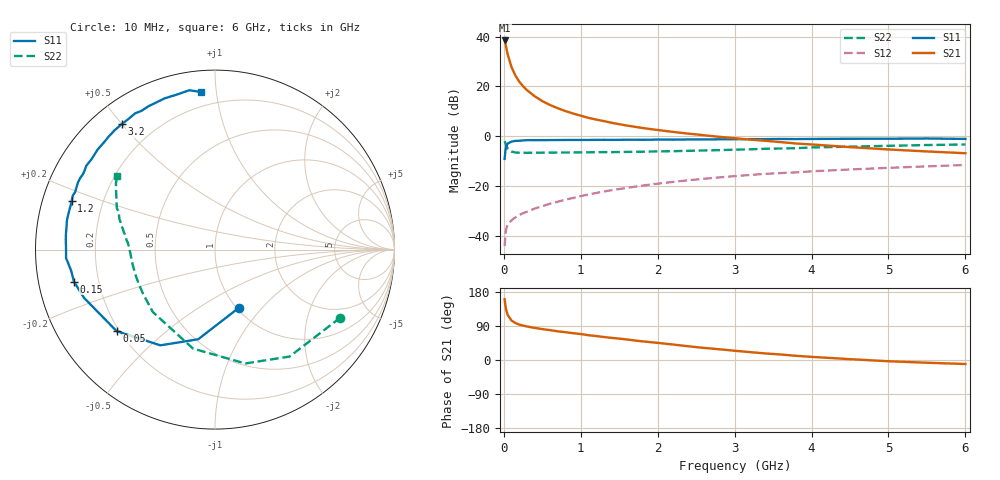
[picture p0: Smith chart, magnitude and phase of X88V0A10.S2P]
! SIEMENS Small Signal Semiconductors
! BFP136W
! Si NPN RF Bipolar Junction Transistor in SOT343
! VCE = 8 V  IC = 100 mA
! Common Emitter S-Parameters:  September  1994
# GHz  S  MA  R  50
!  f  S11  S21  S12  S22
! GHz  MAG  ANG  MAG  ANG  MAG  ANG  MAG  ANG
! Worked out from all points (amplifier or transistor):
!   40 points, 10 MHz to 6 GHz, reference 50 ohm
!   highest |S21| = 38.4 dB at 10 MHz (marker M1)
!   |S21| within 3 dB of that: start of sweep to 31.92 MHz
!   unconditionally stable (mu >= 1): 671.9 MHz to 3.148 GHz
!   at 200 MHz: K = 0.65, MSG = 26.8 dB, |S12| = -31.6 dB
!   at 1.5 GHz: K = 1.10, MAG = 11.1 dB, |S12| = -21.2 dB
!   at 6 GHz: K = 0.96, MSG = 2.4 dB, |S12| = -11.6 dB
!   S11 on the Smith chart (normalised r, x): 10 MHz: 1.02, -0.76; 50 MHz: 0.19, -0.35; 150 MHz: 0.11, -0.11; 1.2 GHz: 0.09, +0.16; 3.2 GHz: 0.09, +0.50; 6 GHz: 0.12, +0.91
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0.01  0.3504 -67.7  83.49 160.6  0.0062 67.8  0.7947 -28.5
0.02  0.5082 -100.6  71.93 144.4  0.0105 59.1  0.7264 -55.1
0.03  0.614 -119.7  61.03 132.8  0.0136 49.7  0.6565 -75.1
0.05  0.7118 -140.3  43.75 118.7  0.0169 40.0  0.565 -102.5
0.1  0.7778 -159.8  24.28 104.0  0.0205 36.8  0.4908 -134.9
0.15  0.8057 -167.2  16.56 97.5  0.0234 39.0  0.4702 -148.6
0.2  0.8096 -171.5  12.47 93.6  0.0262 40.1  0.4657 -156.0
0.25  0.8219 -174.8  10.06 90.7  0.0285 41.8  0.4647 -160.8
0.3  0.8309 -176.7  8.423 88.6  0.0305 43.3  0.4641 -164.0
0.4  0.8302 179.1  6.352 84.7  0.0352 46.3  0.4656 -168.5
0.5  0.8334 176.1  5.066 81.5  0.0394 48.7  0.467 -171.5
0.6  0.8352 173.9  4.227 78.8  0.0441 50.2  0.4686 -173.4
0.7  0.8369 171.1  3.649 75.7  0.0484 52.3  0.4695 -174.9
0.9  0.8406 167.3  2.854 70.7  0.0575 54.1  0.4717 -177.6
1.1  0.8412 163.0  2.334 65.4  0.0675 55.3  0.4751 -179.3
1.2  0.8438 161.3  2.157 63.2  0.0724 55.8  0.4775 179.8
1.7  0.8503 151.9  1.546 51.5  0.0967 55.0  0.4859 175.9
2.2  0.8527 143.6  1.219 40.8  0.1208 52.3  0.5 172.4
3.2  0.8714 126.7  0.853 20.8  0.1665 44.3  0.5453 164.1
4.5  0.8882 108.4  0.603 2.2  0.2147 33.6  0.6171 152.9
5.5  0.8992 99.2  0.494 -7.2  0.2479 25.6  0.6642 146.2
6  0.8813 94.9  0.455 -10.6  0.2642 21.4  0.6814 143.2
